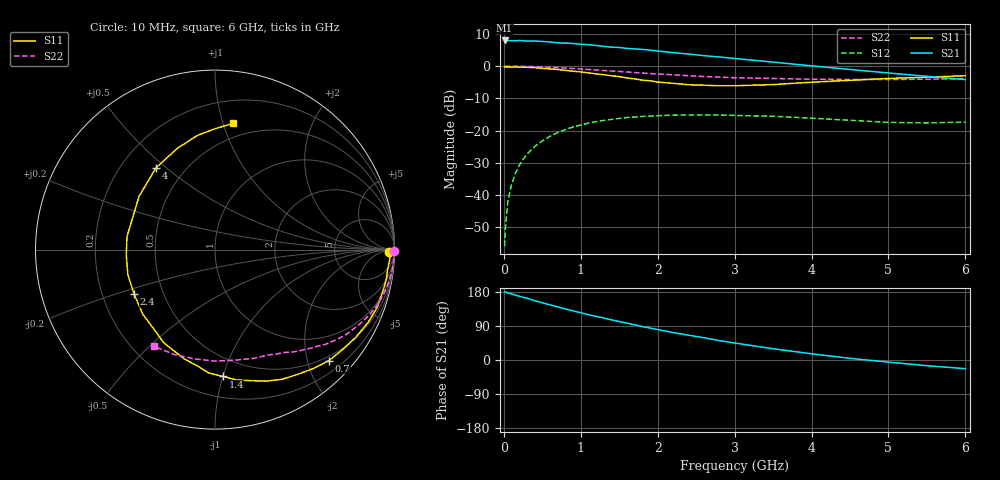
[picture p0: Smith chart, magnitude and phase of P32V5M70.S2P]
! SIEMENS Small Signal Semiconductors
! BFP181
! Si NPN RF Bipolar Junction Transistor in SOT143
! VCE = 2.5 V  IC = 0.7 mA
! Common Emitter S-Parameters:  March  1996
# GHz  S  MA  R  50
!  f  S11  S21  S12  S22
! GHz  MAG  ANG  MAG  ANG  MAG  ANG  MAG  ANG
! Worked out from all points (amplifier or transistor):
!   36 points, 10 MHz to 6 GHz, reference 50 ohm
!   highest |S21| = 8.0 dB at 10 MHz (marker M1)
!   |S21| within 3 dB of that: start of sweep to 1.905 GHz
!   unconditionally stable (mu >= 1): 3.499 GHz to end of sweep
!   at 250 MHz: K = 0.09, MSG = 18.4 dB, |S12| = -29.0 dB
!   at 1.4 GHz: K = 0.45, MSG = 11.2 dB, |S12| = -16.5 dB
!   at 6 GHz: K = 1.37, MAG = 3.0 dB, |S12| = -17.4 dB
!   S11 on the Smith chart (normalised r, x): 10 MHz: 55, -26; 700 MHz: 0.42, -2.40; 1.4 GHz: 0.35, -1.00; 2.4 GHz: 0.34, -0.23; 4 GHz: 0.35, +0.46; 6 GHz: 0.38, +1.07
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0.01  0.9707 -0.8  2.503 179.7  0.0016 82.8  0.9987 -0.3
0.02  0.9743 -1.5  2.479 179.5  0.003 94.5  0.9932 -0.5
0.05  0.9758 -3.0  2.502 177.2  0.0076 91.3  0.997 -1.6
0.1  0.9676 -6.8  2.479 174.3  0.0145 83.9  0.9992 -3.0
0.15  0.9688 -9.6  2.469 171.3  0.0215 82.5  0.995 -4.5
0.25  0.9604 -15.9  2.475 165.5  0.0355 78.9  0.9909 -7.6
0.4  0.9447 -25.4  2.455 156.6  0.0564 72.9  0.9813 -12.0
0.5  0.924 -32.0  2.416 150.9  0.0688 68.0  0.9712 -14.9
0.7  0.8863 -44.2  2.299 140.2  0.0929 59.8  0.9466 -20.5
0.9  0.8331 -56.7  2.246 129.6  0.1136 52.1  0.9178 -25.5
1.1  0.7856 -68.9  2.154 119.5  0.1302 45.0  0.886 -30.3
1.4  0.7079 -86.5  1.97 106.0  0.1488 35.1  0.8399 -36.9
1.5  0.6875 -93.1  1.949 101.5  0.154 32.3  0.8243 -38.6
1.8  0.6064 -112.8  1.815 88.2  0.1652 24.7  0.7807 -43.8
2.2  0.5401 -138.1  1.618 72.4  0.1735 15.2  0.733 -50.4
2.4  0.5142 -151.4  1.541 65.4  0.1743 11.0  0.7101 -53.6
3  0.4956 171.6  1.317 44.8  0.1715 0.8  0.6603 -62.5
3.5  0.5168 145.0  1.154 29.7  0.1666 -5.1  0.6433 -70.3
4  0.562 125.8  1.01 16.4  0.1553 -9.4  0.626 -79.6
4.5  0.6023 110.3  0.887 4.4  0.1442 -11.8  0.6213 -89.8
5.5  0.6736 89.9  0.694 -15.0  0.1315 -7.7  0.627 -111.2
6  0.7095 82.1  0.618 -22.9  0.1348 -4.9  0.6373 -122.3
